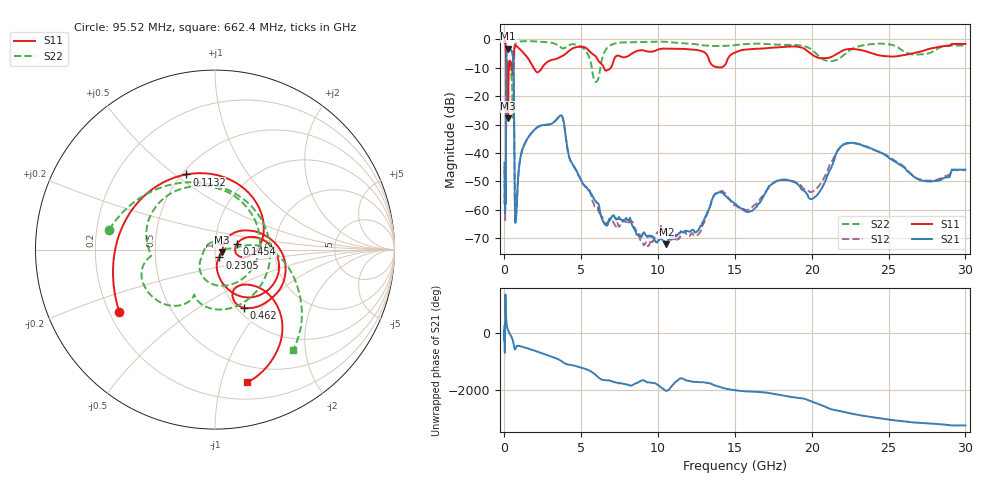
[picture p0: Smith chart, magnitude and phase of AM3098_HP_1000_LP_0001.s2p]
! Date/Time: Thu, Feb 28, 2019 8:39 AM
! Network Analyzer: Agilent Technologies E8364B Rev: A.07.50.67
! Sweep from 0.010 to 30.000 GHz, 1601 Points, Sweep Type: LOG
! Power Supply: 5.022 V, 0.002 A
# Hz S DB R 50
!freq MagS11 AngS11 MagS21 AngS21 MagS12 AngS12 MagS22 AngS22
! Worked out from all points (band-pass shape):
!   1601 points, 10 MHz to 30 GHz, reference 50 ohm
!   highest |S21| = -3.28 dB at 237.5 MHz (marker M1); lowest = -72.1 dB at 10.54 GHz (marker M2)
!   |S21| within 3 dB of the highest: 127.3 MHz to 550.5 MHz (423.2 MHz wide, 125 % of centre)
!   lowest |S11| = -27.8 dB at 236.3 MHz (marker M3), VSWR 1.08, Z = 53.9 - j1.65 ohm
!   |S11| at or under -10 dB: 198.2 MHz to 289.7 MHz (91.47 MHz wide, 37.5 % of centre); 1.898 GHz to 2.442 GHz (543.4 MHz wide, 25 % of centre); 6.475 GHz to 6.92 GHz (445.8 MHz wide, 6.66 % of centre)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
!   |S22| runs from -27.6 to -0.6 dB; largest |S21 - S12| = 0.012
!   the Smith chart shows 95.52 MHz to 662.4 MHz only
!   S11 on the Smith chart (normalised r, x): 95.52 MHz: 0.24, -0.28; 113.2 MHz: 0.53, +0.55; 145.4 MHz: 1.27, +0.08; 230.5 MHz: 1.05, -0.09; 462 MHz: 1.07, -0.80; 662.4 MHz: 0.34, -1.21
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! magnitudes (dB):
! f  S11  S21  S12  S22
! 10 MHz  -0.4  -43.3  -47.1  -0.6
! 38.04 MHz  -0.5  -61.0  -60.7  -0.8
! 95.52 MHz  -3.9  -43.4  -42.0  -4.4
! 113.2 MHz  -7.0  -15.7  -15.7  -10.3
! 144.7 MHz  -18.4  -4.3  -4.3  -10.4
! 145.4 MHz  -18.1  -4.3  -4.2  -10.3
! 188.7 MHz  -8.8  -3.8  -3.8  -7.1
! 230.5 MHz  -26.0  -3.3  -3.3  -8.9
! 236.3 MHz  -27.8  -3.3  -3.3  -8.9
! 237.5 MHz  -27.8  -3.3  -3.3  -8.9
! 462 MHz  -8.8  -4.0  -4.0  -13.3
! 550.5 MHz  -11.8  -6.3  -6.2  -27.3
! 605.4 MHz  -5.6  -15.6  -15.6  -11.6
! 662.4 MHz  -2.4  -51.4  -52.2  -3.0
! 728.5 MHz  -2.1  -63.8  -62.9  -1.3
! 2.084 GHz  -11.4  -31.2  -31.1  -0.7
! 3.704 GHz  -6.0  -26.8  -26.8  -2.9
! 5.959 GHz  -6.0  -57.1  -59.0  -15.0
! 7.926 GHz  -6.1  -62.8  -64.3  -1.0
! 10.54 GHz  -3.2  -72.1  -68.0  -0.9
! 22.56 GHz  -3.4  -36.4  -36.5  -3.5
! 30 GHz  -1.6  -45.9  -46.0  -2.2
